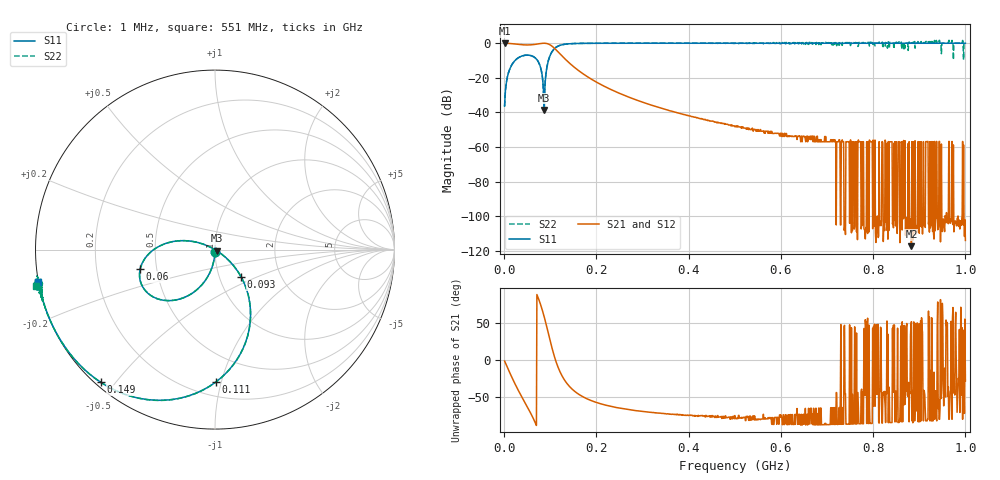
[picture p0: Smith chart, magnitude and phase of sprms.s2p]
# MHz S RI R 50
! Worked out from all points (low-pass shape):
!   999 points, 1 MHz to 1 GHz, reference 50 ohm
!   highest |S21| = 0.00 dB at 1 MHz (marker M1); lowest = -117.3 dB at 883 MHz (marker M2)
!   |S21| within 3 dB of the highest: start of sweep to 109.4 MHz
!   lowest |S11| = -38.5 dB at 87 MHz (marker M3), VSWR 1.02, Z = 51 - j0.649 ohm
!   |S11| at or under -10 dB: start of sweep to 23.59 MHz; 72.36 MHz to 95.97 MHz (23.61 MHz wide, 28 % of centre)
!   |S22| runs from -38.0 to 1.6 dB; largest |S21 - S12| = 0
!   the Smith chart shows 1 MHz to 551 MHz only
!   S11 on the Smith chart (normalised r, x): 1 MHz: 1.00, -0.03; 60 MHz: 0.40, -0.11; 93 MHz: 1.27, -0.41; 111 MHz: 0.30, -0.96; 149 MHz: 0.02, -0.46; 551 MHz: 0.00, -0.09
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1  -0.00039 -0.0153  0.9996 -0.0252  0.9996 -0.0252  -0.000389 -0.0153
18  -0.1087 -0.2298  0.8743 -0.4132  0.8743 -0.4132  -0.1087 -0.2298
60  -0.4165 -0.107  0.2248 -0.8742  0.2248 -0.8742  -0.4162 -0.107
66  -0.3866 -0.0443  0.105 -0.915  0.105 -0.915  -0.3862 -0.0443
75  -0.2731 0.0348  0.1216 0.9534  0.1216 0.9534  -0.2726 0.0347
87  0.01 -0.00636  0.5223 0.8521  0.5223 0.8521  0.0106 -0.00682
93  0.1463 -0.1535  0.706 0.6748  0.706 0.6748  0.1468 -0.1541
111  0.00688 -0.7358  0.6759 0.00681  0.6759 0.00681  0.00682 -0.7366
149  -0.6354 -0.7398  0.1661 -0.1425  0.1661 -0.1425  -0.6358 -0.7402
168  -0.7491 -0.647  0.0914 -0.1057  0.0914 -0.1057  -0.7494 -0.6472
334  -0.9527 -0.303  0.00428 -0.0134  0.00428 -0.0134  -0.9528 -0.3017
502  -0.9799 -0.1989  0.000702 -0.004  0.000702 -0.004  -0.9908 -0.2044
551  -0.9834 -0.1809  0.000477 -0.00316  0.000477 -0.00316  -0.9968 -0.2047
667  -0.9888 -0.149  0.000103 -0.00201  0.000103 -0.00201  -1.022 -0.2082
769  -0.9916 -0.1291  7.7e-05 -0.00142  7.7e-05 -0.00142  -1.024 -0.2195
784  -0.9919 -0.1266  3.23e-06 3.45e-06  3.23e-06 3.45e-06  -1 -2.91e-11
793  -0.9921 -0.1251  8.62e-05 -0.00143  8.62e-05 -0.00143  -1.031 -0.2462
805  -0.9923 -0.1233  3.13e-06 -1.03e-06  3.13e-06 -1.03e-06  -1 0
834  -0.9928 -0.1189  3.11e-06 -2.32e-06  3.11e-06 -2.32e-06  -1 0
883  -0.9936 -0.1123  8.4e-07 1.08e-06  8.4e-07 1.08e-06  -1 0
919  -0.9941 -0.1079  0.000233 -0.00143  0.000233 -0.00143  -1 -0.6667
1000  -0.995 -0.0991  1.77e-06 -9.7e-07  1.77e-06 -9.7e-07  -1 0
